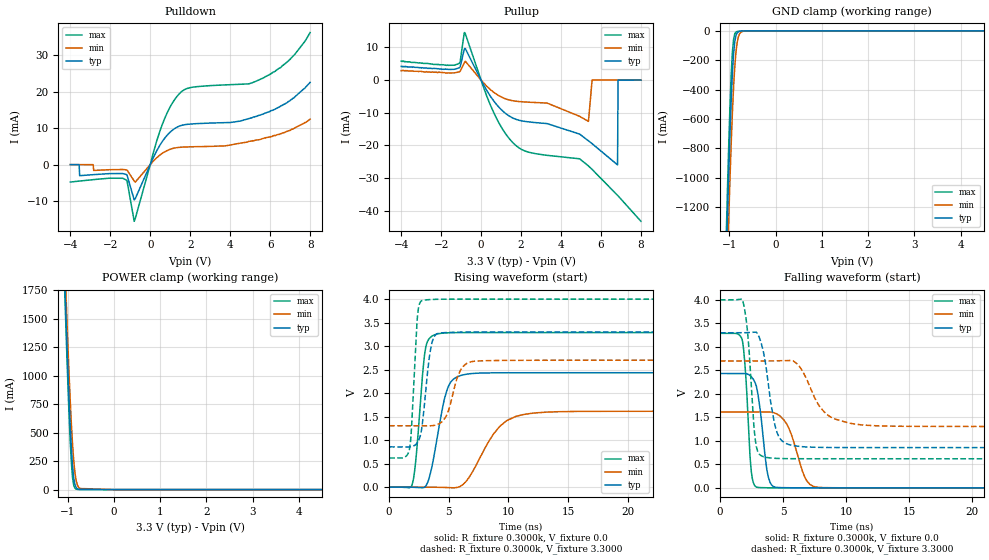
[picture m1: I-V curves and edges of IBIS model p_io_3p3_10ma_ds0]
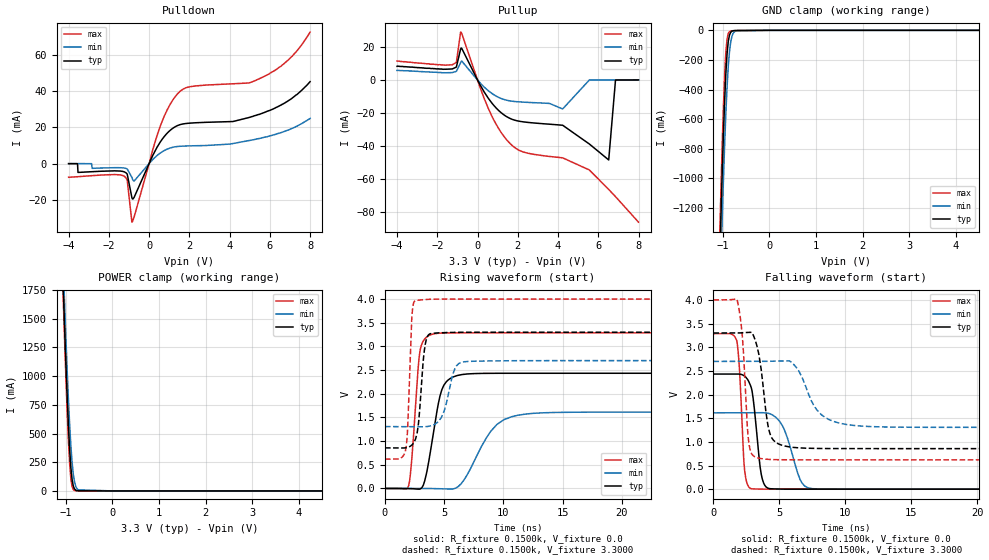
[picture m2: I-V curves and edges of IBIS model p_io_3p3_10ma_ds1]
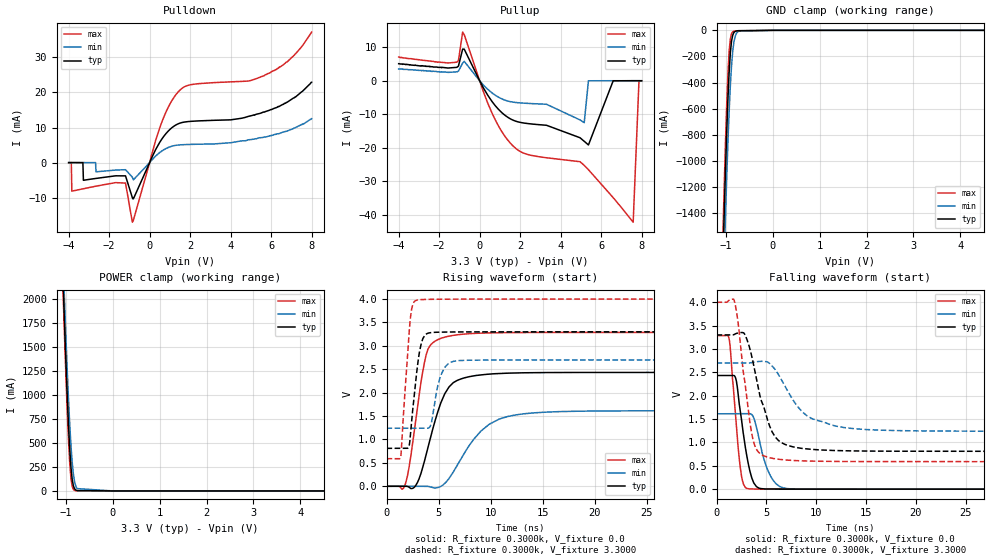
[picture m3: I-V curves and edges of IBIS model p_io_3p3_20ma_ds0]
| IBIS file was generated by Viper version: 2022.06.14
[IBIS Ver]   4.2
[Comment Char]   |_char
[File Name]   ke17z512_64lqfp10x10.ibs
[File Rev]   1
[Date]   Tue Jun 27 20:49:57 2023
[Source]   NXP Viper 2022.06.14
[Notes]
[Disclaimer] IMPORTANT NOTICE
  This information is provided on an AS IS basis and without warranty.
  IN NO EVENT SHALL NXP BE LIABLE FOR INCIDENTAL OR CONSEQUENTIAL
  DAMAGES ARISING FROM USE OF THIS INFORMATION. THIS DISCLAIMER OF
  WARRANTY EXTENDS TO THE USER OF THE INFORMATION, AND TO THEIR CUSTOMERS
  OR USERS OF PRODUCTS  AND IS IN LIEU OF ALL WARRANTIES WHETHER EXPRESS,
  IMPLIED, OR STATUTORY, INCLUDING IMPLIED WARRANTIES OF MERCHANTABILITY
  OR FITNESS FOR PARTICULAR PURPOSE.
  NXP does not represent or warrant that the information furnished
  hereunder is free of infringement of any third party patents,
  copyrights, trade secrets, or other intellectual property rights.
  NXP does not represent or warrant that the information is free of
  defect, or that it meets any particular standard, requirements or need
  of the user of the infomation or their customers.
  NXP reserves the right to change the information in this file
  without notice.
   http://www.nxp.com
[Copyright]   (C) Copyright NXP 2004 - 2023, All Rights Reserved.
|   KE17Z512_64LQFP10x10
[Component]   KE17Z512_64LQFP10x10
[Manufacturer]   NXP
[Package]
| variable   typ   min   max
R_pkg   0.28181   0.17177   0.34309
L_pkg   5.526e-09   4.177e-09   7.456e-09
C_pkg   2.518e-13   2.176e-13   3.261e-13
[Pin] signal_name   model_name   R_pin   L_pin   C_pin
1   PTD1   p_io_20ma_model   0.34309   7.456e-09 2.627e-13
2   PTD0   p_io_20ma_model   0.20185   6.090e-09 3.261e-13
3   PTE11   p_io_5ma_model   0.31644   6.534e-09 2.616e-13
4   PTE10   p_io_5ma_model   0.30709   5.952e-09 2.466e-13
5   PTE5   p_io_5ma_model   0.30545   5.419e-09 2.421e-13
6   PTE4   p_io_5ma_model   0.30549   4.744e-09 2.434e-13
7   VDD   POWER   NA   NA   NA
8   VDDA   POWER   NA   NA   NA
9   VREFH   POWER   0.30507   4.177e-09 2.403e-13
10   VSS   GND   NA   NA   NA
11   PTB7   p_io_5ma_model   0.29864   4.711e-09 2.425e-13
12   PTB6   p_io_5ma_model   0.30074   5.409e-09 2.431e-13
13   PTE3   p_io_5ma_model   0.30315   5.935e-09 2.380e-13
14   PTD16   p_io_20ma_model   0.30605   6.636e-09 2.465e-13
15   PTD15   p_io_20ma_model   0.31779   7.207e-09 2.659e-13
16   PTE9   p_io_5ma_model   0.20325   6.673e-09 3.157e-13
17   PTE8   p_io_5ma_model   0.3128   6.207e-09 2.546e-13
18   PTB5   p_io_20ma_model   0.29863   5.798e-09 2.587e-13
19   PTB4   p_io_20ma_model   0.17608   4.843e-09 3.043e-13
20   PTC3   p_io_5ma_model   0.28307   5.402e-09 2.438e-13
21   PTC2   p_io_5ma_model   0.27909   5.351e-09 2.365e-13
22   PTD7   p_io_5ma_model   0.27794   5.278e-09 2.317e-13
23   PTD6   p_io_5ma_model   0.28016   5.286e-09 2.281e-13
24   PTD5   p_io_5ma_model   0.28599   5.343e-09 2.176e-13
25   PTC1   p_io_5ma_model   0.1779   4.747e-09 2.587e-13
26   PTC0   p_io_5ma_model   0.28246   5.299e-09 2.238e-13
27   PTC17   p_io_5ma_model   0.27878   5.305e-09 2.265e-13
28   PTC16   p_io_5ma_model   0.17177   4.736e-09 2.857e-13
29   PTC15   p_io_5ma_model   0.28065   5.462e-09 2.410e-13
30   PTC14   p_io_5ma_model   0.28686   5.607e-09 2.485e-13
31   PTB3   p_io_5ma_model   0.29762   5.804e-09 2.573e-13
32   PTB2   p_io_10ma_model   0.30999   5.986e-09 2.515e-13
33   PTB1   p_io_5ma_model   0.32395   6.128e-09 2.614e-13
34   PTB0   p_io_5ma_model   0.31088   5.867e-09 2.674e-13
35   PTC9   p_io_5ma_model   0.30054   5.601e-09 2.567e-13
36   PTC8   p_io_5ma_model   0.29612   5.428e-09 2.495e-13
37   PTA7   p_io_5ma_model   0.18073   4.534e-09 2.987e-13
38   PTA6   p_io_5ma_model   0.29648   5.039e-09 2.435e-13
39   PTE7   p_io_5ma_model   0.30202   4.757e-09 2.391e-13
40   VSS   GND   NA   NA   NA
41   VDD   POWER   NA   NA   NA
42   PTB13   p_io_5ma_model   0.29766   5.027e-09 2.268e-13
43   PTB12   p_io_5ma_model   0.29187   5.141e-09 2.398e-13
44   PTD4   p_io_5ma_model   0.28969   5.250e-09 2.428e-13
45   PTD3   p_io_rst_model   0.29067   5.384e-09 2.474e-13
46   PTD2   p_io_5ma_model   0.29615   5.553e-09 2.539e-13
47   PTA3   p_io_5ma_model   0.30586   5.744e-09 2.645e-13
48   PTA2   p_io_5ma_model   0.18938   5.179e-09 3.051e-13
49   PTA1   p_io_5ma_model   0.32424   6.184e-09 2.630e-13
50   PTA0   p_io_5ma_model   0.30932   5.933e-09 2.676e-13
51   PTC7   p_io_5ma_model   0.29708   5.735e-09 2.552e-13
52   PTC6   p_io_5ma_model   0.28924   5.620e-09 2.387e-13
53   PTE6   p_io_5ma_model   0.28943   5.528e-09 2.337e-13
54   PTE2   p_io_5ma_model   0.28547   5.419e-09 2.265e-13
55   PTA13   p_io_5ma_model   0.28938   5.428e-09 2.268e-13
56   PTA12   p_io_5ma_model   0.28981   5.395e-09 2.324e-13
57   PTA11   p_io_5ma_model   0.17781   4.705e-09 2.801e-13
58   PTA10   p_io_5ma_model   0.28108   5.252e-09 2.292e-13
59   PTE1   p_io_20ma_model   0.2773   5.241e-09 2.289e-13
60   PTE0   p_io_20ma_model   0.27701   5.295e-09 2.342e-13
61   PTC5   p_io_5ma_model   0.2798   5.334e-09 2.414e-13
62   PTC4   p_io_5ma_model   0.28663   5.438e-09 2.474e-13
63   PTA5   p_io_rst_model   0.29584   5.588e-09 2.563e-13
64   PTA4   p_io_5ma_model   0.3116   5.917e-09 2.541e-13
[Pin Mapping]   pulldown_ref   pullup_ref
1   VSS   VDD
2   VSS   VDD
3   VSS   VDD
4   VSS   VDD
5   VSS   VDD
6   VSS   VDD
7   NC   VDD
8   NC   VDDA
9   NC   VREFH
10   VSS   NC
11   VSS   VDD
12   VSS   VDD
13   VSS   VDD
14   VSS   VDD
15   VSS   VDD
16   VSS   VDD
17   VSS   VDD
18   VSS   VDD
19   VSS   VDD
20   VSS   VDD
21   VSS   VDD
22   VSS   VDD
23   VSS   VDD
24   VSS   VDD
25   VSS   VDD
26   VSS   VDD
27   VSS   VDD
28   VSS   VDD
29   VSS   VDD
30   VSS   VDD
31   VSS   VDD
32   VSS   VDD
33   VSS   VDD
34   VSS   VDD
35   VSS   VDD
36   VSS   VDD
37   VSS   VDD
38   VSS   VDD
39   VSS   VDD
40   VSS   NC
41   NC   VDD
42   VSS   VDD
43   VSS   VDD
44   VSS   VDD
45   VSS   VDD
46   VSS   VDD
47   VSS   VDD
48   VSS   VDD
49   VSS   VDD
50   VSS   VDD
51   VSS   VDD
52   VSS   VDD
53   VSS   VDD
54   VSS   VDD
55   VSS   VDD
56   VSS   VDD
57   VSS   VDD
58   VSS   VDD
59   VSS   VDD
60   VSS   VDD
61   VSS   VDD
62   VSS   VDD
63   VSS   VDD
64   VSS   VDD
|*   Model Selector   *
[Model Selector] p_io_10ma_model
p_io_3p3_10ma_ds0   half-drive for 3.3v application
p_io_3p3_10ma_ds1   full-drive for 3.3v application
p_io_5p0_10ma_ds0   half-drive for 5.0v application
p_io_5p0_10ma_ds1   full-drive for 5.0v application
[Model Selector] p_io_20ma_model
p_io_3p3_20ma_ds0   half-drive for 3.3v application
p_io_3p3_20ma_ds1   full-drive for 3.3v application
p_io_5p0_20ma_ds0   half-drive for 5.0v application
p_io_5p0_20ma_ds1   full-drive for 5.0v application
[Model Selector] p_io_5ma_model
p_io_3p3_5ma   for 3.3v application
p_io_5p0_5ma   for 5.0v application
[Model Selector] p_io_rst_model
p_io_3p3_rst   for 3.3v application
p_io_5p0_rst   for 5.0v application
| End [Component] MT512X_64LQFP10x10
| Models and submodels in the file (12): p_io_3p3_10ma_ds0 (I/O), p_io_3p3_10ma_ds1 (I/O), p_io_3p3_20ma_ds0 (I/O), p_io_3p3_20ma_ds1 (I/O), p_io_3p3_5ma (I/O), p_io_3p3_rst (I/O), p_io_5p0_10ma_ds0 (I/O), p_io_5p0_10ma_ds1 (I/O), p_io_5p0_20ma_ds0 (I/O), p_io_5p0_20ma_ds1 (I/O), p_io_5p0_5ma (I/O), p_io_5p0_rst (I/O)
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[Model] p_io_3p3_10ma_ds0
|   Model p_io_3p3_10ma_ds0
| This model was characterised for following simulation conditions:
| External (pad) voltage:
|   - Typ: 3.3V,   - Min: 2.7V,   - Max: 4.0V
| Library cells for typ/min/max conditions are connected as defined below:
|  pad - External Pad
|  ipp_do_lv - Core Input
|  ipp_obe_lv - Output Buffer Enable
|  abt_close_nor_rst_mv - vdde
|  dvdd - dvdd
|  dvss - dvss
|  esd_boost - vdde
|  ipp_dse_lv - dvss
|  ipp_ina_280_mv - NC
|  ipp_ina_40_a_mv - NC
|  ipp_ina_40_b_mv - NC
|  ipp_ina_40_c_mv - NC
|  ipp_ina_40_d_mv - NC
|  ipp_ina_40_e_mv - NC
|  ipp_ina_40_f_mv - NC
|  ipp_ina_40_g_mv - NC
|  ipp_ina_40_h_mv - NC
|  ipp_ind_lv - NC
|  ipp_sre_lv - dvss
|  vdde - vdde
|  vsse - vsse
| All other pins connected to ground
Model_type I/O
Polarity   Non-Inverting
Enable   Active-High
Vinl =   0.9900V
Vinh =   2.3100V
Vmeas =  1.6500V
Cref =   50.0000F
C_comp   1.9352pF   1.8468pF   2.0590pF
[Model Spec]
| variable   typ   min   max
Vinh   2.3100V   1.8900V   2.8000V
Vinl   0.9900V   0.8100V   1.2000V
S_overshoot_high   3.6000V   3.0000V   4.3000V
S_overshoot_low   -0.3000V   -0.3000V   -0.3000V
Vmeas   1.6500V   1.3500V   2.0000V
[Temperature Range]   25.0000   0.1250k   -40.0000
[Voltage Range]   3.3000V   2.7000V   4.0000V
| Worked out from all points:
|   slope of the pulldown table from 0 to 0.495 V, typ, clamps not added: 90.9 ohm
|   slope of the pullup table from 0 to 0.495 V, typ, clamps not added: 95.3 ohm
|   rising waveform, R_fixture 0.3000k, V_fixture 0.0: 20-80 % time 1.08ns typ, 2.28ns min, 618ps max; typ from 0 V to 2.43 V
|   rising waveform, R_fixture 0.3000k, V_fixture 3.3000: 20-80 % time 615ps typ, 950ps min, 407ps max; typ from 0.857 V to 3.3 V
|   falling waveform, R_fixture 0.3000k, V_fixture 0.0: 20-80 % time 627ps typ, 1.16ns min, 408ps max; typ from 2.43 V to 0 V
|   falling waveform, R_fixture 0.3000k, V_fixture 3.3000: 20-80 % time 848ps typ, 1.71ns min, 512ps max; typ from 3.3 V to 0.857 V
[Pulldown]
|Voltage   I(typ)   I(min)   I(max)
-4V       0A         10uA       -4.79mA
-3.558V   -10uA      10uA       -4.53mA
-3.532V   -3.04mA    10uA       -4.51mA
-1.166V   -2.774mA   -1.45mA    -4.321mA
-802mV    -9.71mA    -4.496mA   -15.58mA
498mV     5.474mA    2.695mA    9.451mA
1.434V    10.54mA    4.733mA    19.35mA
2.006V    11.15mA    4.894mA    21.17mA
4.944V    12.67mA    6.4mA      22.22mA
5.724V    14.1mA     7.3mA      24mA
6.998V    17.6mA     9.4mA      28.9mA
8V        22.6mA     12.5mA     36.3mA
[Pullup]
|Voltage   I(typ)   I(min)   I(max)
-4V       4.2mA      2.9mA      5.8mA
-1.1V     3.73mA     2.5mA      5.09mA
-814mV    9.683mA    5.577mA    14.47mA
486mV     -5.117mA   -3.013mA   -7.937mA
1.526V    -11.4mA    -6.246mA   -18.7mA
3.3V      -13.29mA   -7.013mA   -23.01mA
4.932V    -16.52mA   -11.08mA   -24.07mA
5.374V    -18.57mA   -12.63mA   -26.26mA
5.556V    -19.44mA   0A         -27.32mA
6.83V     -25.93mA   10uA       -35.25mA
6.856V    -20uA      10uA       -35.42mA
8V        10uA       10uA       -43.19mA
[GND_clamp]
|Voltage   I(typ)   I(min)   I(max)
-4V       -44.22A    -44.15A    -44.31A
-1.062V   -1.538A    -1.84A     -1.36A
-1.036V   -1.238A    -1.547A    -1.053A
-1.01V    -956.2mA   -1.268A    -766.3mA
-958mV    -472.3mA   -768mA     -297.7mA
-932mV    -288.7mA   -557.4mA   -144.7mA
-906mV    -155.5mA   -380.4mA   -57.41mA
-880mV    -73.51mA   -241.5mA   -20.32mA
-828mV    -13.22mA   -77.7mA    -4.19mA
-776mV    -3.062mA   -20.44mA   -2.572mA
-698mV    -1.117mA   -2.814mA   -1.68mA
8V        0A         0A         0A
[POWER_clamp]
|Voltage   I(typ)   I(min)   I(max)
-4V       44.89A     44.69A     45.07A
-1.074V   1.999A     2.184A     1.905A
-1.048V   1.679A     1.877A     1.575A
-1.022V   1.371A     1.58A      1.256A
-970mV    807.7mA    1.033A     674.4mA
-918mV    359.9mA    574.8mA    234.3mA
-892mV    203mA      392.8mA    103.5mA
-866mV    99.48mA    249.2mA    36.93mA
-814mV    17.16mA    79.21mA    3.9mA
-736mV    1.301mA    9.822mA    753.1uA
0V        71.73pA    1.381nA    67.44pA
8V        0A         0A         0A
[Ramp]
| variable   typ   min   max
dV/dt_r  1.4602/1.0838n   0.9683/2.2799n   1.9729/0.6182n
dV/dt_f  1.4660/0.8478n   0.8362/1.7102n   2.0284/0.5117n
R_load = 0.3000k
[Rising Waveform]
R_fixture= 0.3000k
V_fixture= 0.0
V_fixture_min= 0.0
V_fixture_max= 0.0
|time   V(typ)   V(min)   V(max)
0s        106.2pV    30.82nV    370.3pV
1.909ns   -2.548mV   95.37uV    37.55mV
2.282ns   -5.975mV   129.3uV    694.4mV
2.976ns   278.7uV    -25.48uV   2.834V
3.937ns   915.6mV    -2.42mV    3.253V
4.997ns   2.162V     -10.87mV   3.284V
6.36ns    2.398V     98.12mV    3.288V
9.264ns   2.433V     1.29V      3.288V
11.18ns   2.433V     1.54V      3.288V
40ns      2.434V     1.614V     3.288V
[Rising Waveform]
R_fixture= 0.3000k
V_fixture= 3.3000
V_fixture_min= 2.7000
V_fixture_max= 4.0000
|time   V(typ)   V(min)   V(max)
0s        856.6mV    1.306V     619.2mV
1.701ns   855.8mV    1.306V     804.6mV
1.845ns   860.9mV    1.306V     1.138V
2.381ns   951.8mV    1.304V     3.651V
2.747ns   1.277V     1.303V     3.968V
3.475ns   2.937V     1.304V     3.992V
4.151ns   3.274V     1.344V     3.998V
5.997ns   3.297V     2.494V     4V
7.08ns    3.299V     2.677V     4V
40ns      3.3V       2.7V       4V
[Falling Waveform]
R_fixture= 0.3000k
V_fixture= 0.0
V_fixture_min= 0.0
V_fixture_max= 0.0
|time   V(typ)   V(min)   V(max)
0s        2.434V     1.614V     3.288V
1.753ns   2.435V     1.614V     3.162V
2.02ns    2.432V     1.614V     2.481V
2.489ns   2.365V     1.613V     339.9mV
2.969ns   2.058V     1.614V     10.45mV
3.738ns   356.5mV    1.616V     1.96mV
4.358ns   16.63mV    1.59V      786.2uV
6.904ns   417.9uV    142.8mV    43.92uV
7.622ns   203.8uV    17.7mV     25.27uV
40ns      2.749uV    5.689uV    1.304uV
[Falling Waveform]
R_fixture= 0.3000k
V_fixture= 3.3000
V_fixture_min= 2.7000
V_fixture_max= 4.0000
|time   V(typ)   V(min)   V(max)
0s        3.3V       2.7V       4V
1.8ns     3.3V       2.7V       3.986V
2.189ns   3.304V     2.7V       3.316V
2.792ns   3.313V     2.7V       1.037V
3.465ns   2.866V     2.7V       662.3mV
4.501ns   1.197V     2.704V     626.7mV
5.681ns   906.7mV    2.708V     620.5mV
8.425ns   859.6mV    1.574V     619.3mV
10.78ns   857.1mV    1.354V     619.3mV
40ns      856.6mV    1.306V     619.3mV
[Model] p_io_3p3_10ma_ds1
|   Model p_io_3p3_10ma_ds1
| This model was characterised for following simulation conditions:
| External (pad) voltage:
|   - Typ: 3.3V,   - Min: 2.7V,   - Max: 4.0V
| Library cells for typ/min/max conditions are connected as defined below:
|  pad - External Pad
|  ipp_do_lv - Core Input
|  ipp_obe_lv - Output Buffer Enable
|  abt_close_nor_rst_mv - vdde
|  dvdd - dvdd
|  dvss - dvss
|  esd_boost - vdde
|  ipp_dse_lv - dvdd
|  ipp_ina_280_mv - NC
|  ipp_ina_40_a_mv - NC
|  ipp_ina_40_b_mv - NC
|  ipp_ina_40_c_mv - NC
|  ipp_ina_40_d_mv - NC
|  ipp_ina_40_e_mv - NC
|  ipp_ina_40_f_mv - NC
|  ipp_ina_40_g_mv - NC
|  ipp_ina_40_h_mv - NC
|  ipp_ind_lv - NC
|  ipp_sre_lv - dvss
|  vdde - vdde
|  vsse - vsse
| All other pins connected to ground
Model_type I/O
Polarity   Non-Inverting
Enable   Active-High
Vinl =   0.9900V
Vinh =   2.3100V
Vmeas =  1.6500V
Cref =   50.0000F
C_comp   1.9352pF   1.8468pF   2.0590pF
[Model Spec]
| variable   typ   min   max
Vinh   2.3100V   1.8900V   2.8000V
Vinl   0.9900V   0.8100V   1.2000V
S_overshoot_high   3.6000V   3.0000V   4.3000V
S_overshoot_low   -0.3000V   -0.3000V   -0.3000V
Vmeas   1.6500V   1.3500V   2.0000V
[Temperature Range]   25.0000   0.1250k   -40.0000
[Voltage Range]   3.3000V   2.7000V   4.0000V
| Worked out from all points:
|   slope of the pulldown table from 0 to 0.495 V, typ, clamps not added: 45.6 ohm
|   slope of the pullup table from 0 to 0.495 V, typ, clamps not added: 47.9 ohm
|   rising waveform, R_fixture 0.1500k, V_fixture 0.0: 20-80 % time 1ns typ, 2.22ns min, 557ps max; typ from 0 V to 2.43 V
|   rising waveform, R_fixture 0.1500k, V_fixture 3.3000: 20-80 % time 464ps typ, 836ps min, 293ps max; typ from 0.857 V to 3.3 V
|   falling waveform, R_fixture 0.1500k, V_fixture 0.0: 20-80 % time 535ps typ, 1.09ns min, 340ps max; typ from 2.43 V to 0 V
|   falling waveform, R_fixture 0.1500k, V_fixture 3.3000: 20-80 % time 671ps typ, 1.53ns min, 418ps max; typ from 3.3 V to 0.857 V
[Pulldown]
|Voltage   I(typ)   I(min)   I(max)
-4V       0A         10uA       -7.52mA
-3.558V   -30uA      10uA       -7.21mA
-3.532V   -4.85mA    20uA       -7.19mA
-1.218V   -4.599mA   -2.451mA   -7.053mA
-1.088V   -5.751mA   -2.907mA   -9.093mA
-854mV    -18.79mA   -7.618mA   -32.27mA
-750mV    -18.71mA   -9.652mA   -29.65mA
550mV     11.84mA    5.811mA    20.5mA
1.434V    21.07mA    9.466mA    38.7mA
5.464V    27.1mA     13.8mA     46.72mA
6.894V    34.5mA     18.4mA     56.9mA
8V        45.2mA     24.9mA     72.5mA
[Pullup]
|Voltage   I(typ)   I(min)   I(max)
-4V       8.3mA      5.8mA      11.5mA
-1.256V   6.69mA     4.49mA     9.21mA
-1.048V   8.03mA     5.34mA     11mA
-814mV    19.34mA    11.14mA    28.9mA
538mV     -11.14mA   -6.546mA   -17.3mA
1.552V    -22.94mA   -12.55mA   -37.69mA
2.332V    -25.48mA   -13.47mA   -43.87mA
4.23V     -27.44mA   -17.57mA   -47.21mA
5.556V    -38.82mA   -10uA      -54.56mA
6.518V    -48.48mA   10uA       -66.38mA
6.856V    -30uA      20uA       -70.73mA
8V        30uA       20uA       -86.22mA
[GND_clamp]
|Voltage   I(typ)   I(min)   I(max)
-4V       -44.22A    -44.15A    -44.31A
-1.062V   -1.538A    -1.84A     -1.36A
-1.036V   -1.238A    -1.547A    -1.053A
-1.01V    -956.2mA   -1.268A    -766.3mA
-958mV    -472.3mA   -768mA     -297.7mA
-932mV    -288.7mA   -557.4mA   -144.7mA
-906mV    -155.5mA   -380.4mA   -57.41mA
-880mV    -73.51mA   -241.5mA   -20.32mA
-828mV    -13.22mA   -77.7mA    -4.19mA
-776mV    -3.062mA   -20.44mA   -2.572mA
-698mV    -1.117mA   -2.814mA   -1.68mA
8V        0A         0A         0A
[POWER_clamp]
|Voltage   I(typ)   I(min)   I(max)
-4V       44.89A     44.69A     45.07A
-1.074V   1.999A     2.184A     1.905A
-1.048V   1.679A     1.877A     1.575A
-1.022V   1.371A     1.58A      1.256A
-970mV    807.7mA    1.033A     674.4mA
-918mV    359.9mA    574.8mA    234.3mA
-892mV    203mA      392.8mA    103.5mA
-866mV    99.48mA    249.2mA    36.93mA
-814mV    17.16mA    79.21mA    3.9mA
-736mV    1.301mA    9.822mA    753.1uA
0V        71.73pA    1.381nA    67.44pA
8V        0A         0A         0A
[Ramp]
| variable   typ   min   max
dV/dt_r  1.4597/1.0002n   0.9678/2.2159n   1.9721/0.5574n
dV/dt_f  1.4659/0.6708n   0.8362/1.5330n   2.0283/0.4180n
R_load = 0.1500k
[Rising Waveform]
R_fixture= 0.1500k
V_fixture= 0.0
V_fixture_min= 0.0
V_fixture_max= 0.0
|time   V(typ)   V(min)   V(max)
0s        55.35pV    15.57nV    185.3pV
2.002ns   -2.948mV   65.27uV    58.54mV
2.256ns   -4.984mV   79.5uV     588.3mV
2.942ns   -13.11mV   -15.13uV   2.877V
3.908ns   884.5mV    -2.158mV   3.251V
4.803ns   2.085V     -7.521mV   3.282V
6.48ns    2.404V     115.1mV    3.287V
8.94ns    2.432V     1.209V     3.287V
11.22ns   2.433V     1.546V     3.287V
40ns      2.433V     1.613V     3.287V
[Rising Waveform]
R_fixture= 0.1500k
V_fixture= 3.3000
V_fixture_min= 2.7000
V_fixture_max= 4.0000
|time   V(typ)   V(min)   V(max)
0s        856.8mV    1.306V     619.5mV
1.794ns   859.6mV    1.305V     877.7mV
1.919ns   866.8mV    1.305V     1.287V
2.255ns   912.3mV    1.304V     3.54V
2.573ns   1.038V     1.303V     3.966V
2.833ns   1.376V     1.302V     3.977V
3.334ns   2.929V     1.303V     3.989V
3.895ns   3.272V     1.324V     3.996V
6.721ns   3.299V     2.677V     4V
40ns      3.3V       2.7V       4V
[Falling Waveform]
R_fixture= 0.1500k
V_fixture= 0.0
V_fixture_min= 0.0
V_fixture_max= 0.0
|time   V(typ)   V(min)   V(max)
0s        2.433V     1.613V     3.287V
1.79ns    2.435V     1.613V     3.116V
1.986ns   2.433V     1.613V     2.5V
2.371ns   2.387V     1.613V     391.2mV
2.894ns   2.122V     1.613V     8.181mV
3.619ns   328mV      1.616V     1.628mV
4.253ns   11.48mV    1.595V     592.8uV
5.209ns   2.075mV    1.354V     145.2uV
7.312ns   180.5uV    18.48mV    16.22uV
40ns      1.359uV    2.761uV    626.3nV
[Falling Waveform]
R_fixture= 0.1500k
V_fixture= 3.3000
V_fixture_min= 2.7000
V_fixture_max= 4.0000
|time   V(typ)   V(min)   V(max)
0s        3.3V       2.7V       4V
1.796ns   3.3V       2.7V       4.003V
2.214ns   3.305V     2.7V       3.168V
2.649ns   3.313V     2.7V       1.068V
3.301ns   3.028V     2.7V       667.3mV
4.282ns   1.178V     2.703V     627.8mV
5.61ns    900.1mV    2.711V     620.4mV
7.851ns   860.6mV    1.671V     619.6mV
10.07ns   857.3mV    1.367V     619.5mV
40ns      856.8mV    1.306V     619.5mV
[Model] p_io_3p3_20ma_ds0
|   Model p_io_3p3_20ma_ds0
| This model was characterised for following simulation conditions:
| External (pad) voltage:
|   - Typ: 3.3V,   - Min: 2.7V,   - Max: 4.0V
| Library cells for typ/min/max conditions are connected as defined below:
|  pad - External Pad
|  ipp_do_lv - Core Input
|  ipp_obe_lv - Output Buffer Enable
|  abt_close_nor_rst_mv - vdde
|  dvdd - dvdd
|  dvss - dvss
|  esd_boost - vdde
|  ipp_dse_lv - dvss
|  ipp_ina_280_mv - NC
|  ipp_ina_40_a_mv - NC
|  ipp_ina_40_b_mv - NC
|  ipp_ina_40_c_mv - NC
|  ipp_ina_40_d_mv - NC
|  ipp_ina_40_e_mv - NC
|  ipp_ina_40_f_mv - NC
|  ipp_ina_40_g_mv - NC
|  ipp_ina_40_h_mv - NC
|  ipp_ind_lv - NC
|  vdde - vdde
|  vsse - vsse
| All other pins connected to ground
Model_type I/O
Polarity   Non-Inverting
Enable   Active-High
Vinl =   0.9900V
Vinh =   2.3100V
Vmeas =  1.6500V
Cref =   50.0000F
C_comp   2.8325pF   2.6979pF   3.0285pF
[Model Spec]
| variable   typ   min   max
Vinh   2.3100V   1.8900V   2.8000V
Vinl   0.9900V   0.8100V   1.2000V
S_overshoot_high   3.6000V   3.0000V   4.3000V
S_overshoot_low   -0.3000V   -0.3000V   -0.3000V
Vmeas   1.6500V   1.3500V   2.0000V
[Temperature Range]   25.0000   0.1250k   -40.0000
[Voltage Range]   3.3000V   2.7000V   4.0000V
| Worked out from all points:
|   slope of the pulldown table from 0 to 0.495 V, typ, clamps not added: 86.1 ohm
|   slope of the pullup table from 0 to 0.495 V, typ, clamps not added: 95.9 ohm
|   rising waveform, R_fixture 0.3000k, V_fixture 0.0: 20-80 % time 1.95ns typ, 3.22ns min, 1.29ns max; typ from 0 V to 2.43 V
|   rising waveform, R_fixture 0.3000k, V_fixture 3.3000: 20-80 % time 737ps typ, 841ps min, 627ps max; typ from 0.81 V to 3.3 V
|   falling waveform, R_fixture 0.3000k, V_fixture 0.0: 20-80 % time 1.03ns typ, 1.28ns min, 774ps max; typ from 2.43 V to 0 V
|   falling waveform, R_fixture 0.3000k, V_fixture 3.3000: 20-80 % time 1.83ns typ, 3.04ns min, 1.16ns max; typ from 3.3 V to 0.81 V
[Pulldown]
|Voltage   I(typ)   I(min)   I(max)
-4V       10uA       10uA       -80uA
-3.87V    10uA       10uA       -90uA
-3.844V   0A         10uA       -8.14mA
-3.298V   -10uA      0A         -7.48mA
-3.272V   -5.04mA    10uA       -7.45mA
-1.192V   -3.779mA   -2.025mA   -5.84mA
-854mV    -10mA      -4.159mA   -16.99mA
498mV     5.783mA    2.872mA    9.907mA
1.434V    11.11mA    5.018mA    20.3mA
5.672V    14.4mA     7.3mA      24.8mA
6.79V     17.2mA     9mA        28.7mA
8V        22.9mA     12.5mA     37.2mA
[Pullup]
|Voltage   I(typ)   I(min)   I(max)
-4V       5.1mA      3.5mA      7.1mA
-1.126V   4.01mA     2.66mA     5.55mA
-840mV    9.451mA    5.276mA    14.53mA
616mV     -6.231mA   -3.647mA   -9.711mA
1.526V    -11.39mA   -6.242mA   -18.68mA
3.3V      -13.28mA   -7.01mA    -22.99mA
5.166V    -18.07mA   -12.5mA    -25.25mA
5.374V    -19.16mA   0A         -26.55mA
6.596V    -10uA      10uA       -34.89mA
7.584V    20uA       10uA       -42.22mA
7.87V     20uA       10uA       -90uA
8V        20uA       0A         -80uA
[GND_clamp]
|Voltage   I(typ)   I(min)   I(max)
-4V       -49.59A    -49.54A    -49.68A
-1.062V   -1.74A     -2.082A    -1.538A
-1.036V   -1.402A    -1.75A     -1.192A
-1.01V    -1.083A    -1.435A    -869.2mA
-984mV    -791.3mA   -1.14A     -579.3mA
-958mV    -535mA     -869mA     -338.2mA
-932mV    -326.2mA   -629.6mA   -164.5mA
-906mV    -175.2mA   -428.2mA   -66.24mA
-880mV    -83.05mA   -270.6mA   -25.06mA
-828mV    -16.12mA   -86.77mA   -7.14mA
-724mV    -2.673mA   -6.605mA   -3.909mA
8V        0A         0A         0A
[POWER_clamp]
|Voltage   I(typ)   I(min)   I(max)
-4V       52.67A     52.45A     52.88A
-1.074V   2.381A     2.6A       2.272A
-1.048V   2.004A     2.236A     1.882A
-1.022V   1.639A     1.885A     1.505A
-970mV    970.2mA    1.235A     814mA
-918mV    434.5mA    688.7mA    285.8mA
-892mV    245.5mA    470.7mA    127mA
-866mV    120.4mA    298.4mA    45.78mA
-814mV    21.03mA    94.6mA     5.402mA
-762mV    3.719mA    24.12mA    1.768mA
0V        97.57pA    2.637nA    84.84pA
8V        0A         0A         0A
[Ramp]
| variable   typ   min   max
dV/dt_r  1.4597/1.9485n   0.9680/3.2184n   1.9722/1.2863n
dV/dt_f  1.4937/1.8347n   0.8757/3.0424n   2.0462/1.1640n
R_load = 0.3000k
[Rising Waveform]
R_fixture= 0.3000k
V_fixture= 0.0
V_fixture_min= 0.0
V_fixture_max= 0.0
|time   V(typ)   V(min)   V(max)
0s        178.7pV    57.84nV    702.6pV
1.772ns   270.5uV    7.879uV    25.56mV
2.267ns   -37.08mV   38.7uV     544.7mV
2.8ns     15.36mV    60.05uV    1.413V
3.8ns     671mV      305uV      2.804V
5.289ns   1.823V     8.293mV    3.166V
6.762ns   2.259V     440.3mV    3.236V
9.056ns   2.38V      1.178V     3.272V
11.65ns   2.417V     1.492V     3.283V
40ns      2.433V     1.613V     3.287V
[Rising Waveform]
R_fixture= 0.3000k
V_fixture= 3.3000
V_fixture_min= 2.7000
V_fixture_max= 4.0000
|time   V(typ)   V(min)   V(max)
0s        810.5mV    1.24V      589.7mV
1.359ns   811mV      1.241V     631.1mV
2.243ns   972.4mV    1.241V     3.49V
2.849ns   2.336V     1.241V     3.974V
3.173ns   2.885V     1.241V     3.986V
3.673ns   3.226V     1.241V     3.992V
4.259ns   3.283V     1.315V     3.995V
5.42ns    3.294V     2.472V     3.998V
6.6ns     3.297V     2.676V     3.999V
40ns      3.3V       2.7V       4V
[Falling Waveform]
R_fixture= 0.3000k
V_fixture= 0.0
V_fixture_min= 0.0
V_fixture_max= 0.0
|time   V(typ)   V(min)   V(max)
0s        2.433V     1.613V     3.287V
1.269ns   2.433V     1.613V     3.21V
1.936ns   2.364V     1.613V     1.47V
2.336ns   1.743V     1.613V     539.3mV
2.577ns   1.365V     1.613V     198.1mV
3.013ns   741.9mV    1.614V     19.2mV
3.986ns   57.14mV    1.339V     2.778mV
5.229ns   3.199mV    363.1mV    1.159mV
6.69ns    1.209mV    27.32mV    489.7uV
40ns      216.1nV    659.8nV    94.46nV
[Falling Waveform]
R_fixture= 0.3000k
V_fixture= 3.3000
V_fixture_min= 2.7000
V_fixture_max= 4.0000
|time   V(typ)   V(min)   V(max)
0s        3.3V       2.7V       4V
1.797ns   3.313V     2.7V       4.022V
2.777ns   3.333V     2.7V       2.385V
3.623ns   2.756V     2.714V     1.09V
4.93ns    1.617V     2.73V      698.5mV
5.881ns   1.118V     2.562V     650.4mV
6.789ns   964.5mV    2.235V     626.9mV
9.121ns   859.6mV    1.562V     602.4mV
12.21ns   824.9mV    1.339V     593mV
40ns      810.5mV    1.24V      589.7mV
